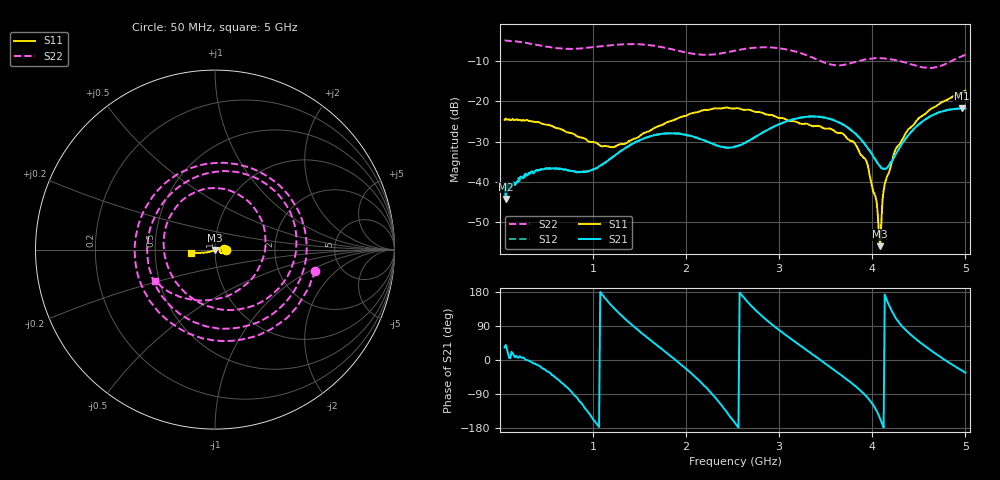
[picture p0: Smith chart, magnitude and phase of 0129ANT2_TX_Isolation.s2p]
! MASWSS0129 de-embedded Sparameters using port extention method. ANT2 to TX Isolation using 3 volt control
! 100pF blocking capacitor
! Sample board 1000013136
# Hz  S  DB  R  50
! Freq  S11  S21  S12  S22
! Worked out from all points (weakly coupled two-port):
!   401 points, 50 MHz to 5 GHz, reference 50 ohm
!   highest |S21| = -21.73 dB at 4.963 GHz (marker M1); lowest = -44.2 dB at 62.38 MHz (marker M2)
!   lowest |S11| = -55.9 dB at 4.084 GHz (marker M3), VSWR 1.00, Z = 50 - j0.154 ohm
!   |S11| at or under -10 dB: start of sweep to end of sweep
!   |S22| runs from -11.7 to -4.9 dB; largest |S21 - S12| = 0.0059
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5e7  -24.58 -3.3  -40.75 33.2  -42.80 50.3  -4.90 -11.9
6.2375e7  -24.24 -1.7  -44.22 39.8  -40.75 0.0  -4.91 -14.8
4.08875e8  -25.14 -18.6  -37.09 -14.1  -37.19 -14.2  -6.02 -97.9
6.44e8  -26.75 -26.7  -36.66 -56.0  -36.58 -55.6  -6.86 -158.0
8.79125e8  -28.96 -30.6  -37.52 -115.1  -37.54 -115.4  -6.87 142.6
1.12663e9  -31.04 -18.3  -35.18 163.2  -35.25 164.3  -6.24 82.1
1.3865e9  -29.80 11.4  -31.07 99.0  -31.01 98.6  -5.81 22.4
1.70825e9  -26.12 25.4  -28.19 34.8  -28.14 34.5  -6.41 -51.0
1.90625e9  -24.26 20.2  -27.94 -4.0  -27.99 -4.7  -7.40 -99.8
2.14138e9  -22.52 11.2  -29.27 -54.7  -29.24 -55.0  -8.38 -163.5
2.525e9  -21.72 -0.3  -31.19 -166.2  -31.20 -166.3  -7.42 97.6
2.95813e9  -23.76 -4.7  -26.07 86.5  -26.08 86.4  -6.72 12.3
3.35413e9  -26.11 4.7  -23.69 15.3  -23.74 15.6  -9.11 -74.1
3.60163e9  -27.56 14.3  -24.85 -28.4  -24.80 -28.7  -11.04 -148.5
3.812e9  -30.38 16.7  -27.92 -68.0  -27.90 -68.1  -10.25 148.5
3.94813e9  -35.58 16.7  -31.54 -99.5  -31.45 -99.4  -9.52 117.2
4.08425e9  -55.89 -106.7  -36.05 -155.0  -36.18 -154.7  -9.31 89.0
4.18325e9  -37.35 -148.4  -35.73 143.1  -35.84 142.1  -9.51 68.3
4.505e9  -24.06 -164.0  -25.63 47.9  -25.63 48.1  -11.40 -12.7
4.72775e9  -20.51 -169.2  -22.59 8.9  -22.64 8.1  -11.30 -85.2
4.96288e9  -17.79 -172.0  -21.73 -27.6  -21.77 -28.2  -8.79 -145.5
5e9  -17.37 -171.9  -21.75 -33.4  -21.79 -33.9  -8.45 -152.5
